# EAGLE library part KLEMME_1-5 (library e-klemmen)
Klemme 5 Pol.
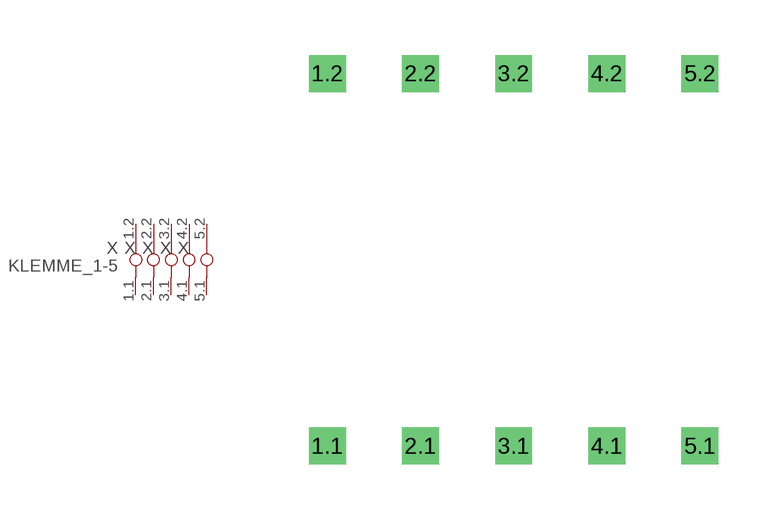
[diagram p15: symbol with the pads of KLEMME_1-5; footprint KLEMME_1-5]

Designator prefix X; gates 1=KLEMME_1-1 2=KLEMME_2 3=KLEMME_3 4=KLEMME_4 5=KLEMME_5

## KLEMME_1-5  [KLEMME_1-5]
1.1  1:1.1  pas
1.2  1:1.2  pas
2.1  2:2.1  pas
2.2  2:2.2  pas
3.1  3:3.1  pas
3.2  3:3.2  pas
4.1  4:4.1  pas
4.2  4:4.2  pas
5.1  5:5.1  pas
5.2  5:5.2  pas

## Footprint KLEMME_1-5 (pad centres in mm)
Dummy
drill 0.5 pad 1 square: 1.1 0,-12.7; 1.2 0,-2.54; 2.1 2.54,-12.7; 2.2 2.54,-2.54; 3.1 5.08,-12.7; 3.2 5.08,-2.54; 4.1 7.62,-12.7; 4.2 7.62,-2.54; 5.1 10.16,-12.7; 5.2 10.16,-2.54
